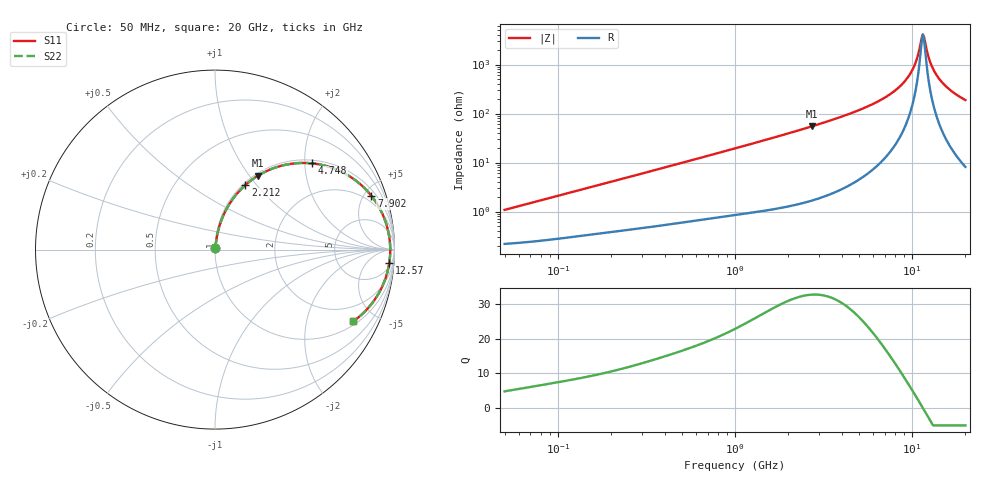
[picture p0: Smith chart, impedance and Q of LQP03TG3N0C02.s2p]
!Murata Part Number: LQP03TG3N0C02
!These Parameters are Measured in Series Mode Connection
!  o--[Z]--o
!Port1  Port2
!  o-------o
!Freq. Start=50[MHz] Stop=20[GHz], 401[Steps]
# Hz S RI R 50
!Freq.(Hz) S11(Real) S11(Imag) S21(Real) S21(Imag) S12(Real) S12(Imag) S22(Real) S22(Imag)
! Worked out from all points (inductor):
!   401 points, 50 MHz to 20 GHz, reference 50 ohm
!   read as one part in series: L = 3.36 nH near 51.52 MHz
!   highest Q = 32.8 at 2.728 GHz (marker M1), where L = 3.22 nH
!   self-resonance near 11.49 GHz
!   S11 on the Smith chart (normalised r, x): 50 MHz: 1.00, +0.02; 2.212 GHz: 1.03, +0.88; 4.748 GHz: 1.08, +2.18; 7.902 GHz: 1.42, +5.65; 12.57 GHz: 8, -23; 20 GHz: 1.16, -3.77
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5e7  0.00229 0.0106  0.9977 -0.0106  0.9977 -0.0106  0.00229 0.0106
1.364002e8  0.00398 0.0278  0.996 -0.0278  0.996 -0.0278  0.00398 0.0278
3.721004e8  0.0104 0.0726  0.9896 -0.0726  0.9896 -0.0726  0.0104 0.0726
1e9  0.044 0.1844  0.956 -0.1844  0.956 -0.1844  0.044 0.1844
2.211938e9  0.1691 0.3595  0.8309 -0.3595  0.8309 -0.3595  0.1691 0.3595
2.728004e9  0.2399 0.4121  0.7601 -0.4121  0.7601 -0.4121  0.2399 0.4121
4.748272e9  0.5412 0.4804  0.4588 -0.4804  0.4588 -0.4804  0.5412 0.4804
6.125241e9  0.7162 0.4279  0.2838 -0.4279  0.2838 -0.4279  0.7162 0.4279
7.442007e9  0.8393 0.336  0.1607 -0.336  0.1607 -0.336  0.8393 0.336
7.901521e9  0.8719 0.2989  0.1281 -0.2989  0.1281 -0.2989  0.8719 0.2989
9.041845e9  0.9312 0.2025  0.0688 -0.2025  0.0688 -0.2025  0.9312 0.2025
9.892087e9  0.958 0.1303  0.042 -0.1303  0.042 -0.1303  0.958 0.1303
1.050288e10  0.9695 0.0798  0.0305 -0.0798  0.0305 -0.0798  0.9695 0.0798
1.115139e10  0.9755 0.0282  0.0245 -0.0282  0.0245 -0.0282  0.9755 0.0282
1.149051e10  0.9764 0.00221  0.0236 -0.00221  0.0236 -0.00221  0.9764 0.00221
1.166392e10  0.9763 -0.0108  0.0237 0.0108  0.0237 0.0108  0.9763 -0.0108
1.183995e10  0.9759 -0.0238  0.0241 0.0238  0.0241 0.0238  0.9759 -0.0238
1.257102e10  0.9708 -0.0756  0.0292 0.0756  0.0292 0.0756  0.9708 -0.0756
1.354865e10  0.9568 -0.1389  0.0432 0.1389  0.0432 0.1389  0.9568 -0.1389
1.482269e10  0.9293 -0.211  0.0707 0.211  0.0707 0.211  0.9293 -0.211
1.696185e10  0.8688 -0.3071  0.1312 0.3071  0.1312 0.3071  0.8688 -0.3071
2e10  0.7713 -0.3989  0.2287 0.3989  0.2287 0.3989  0.7713 -0.3989
